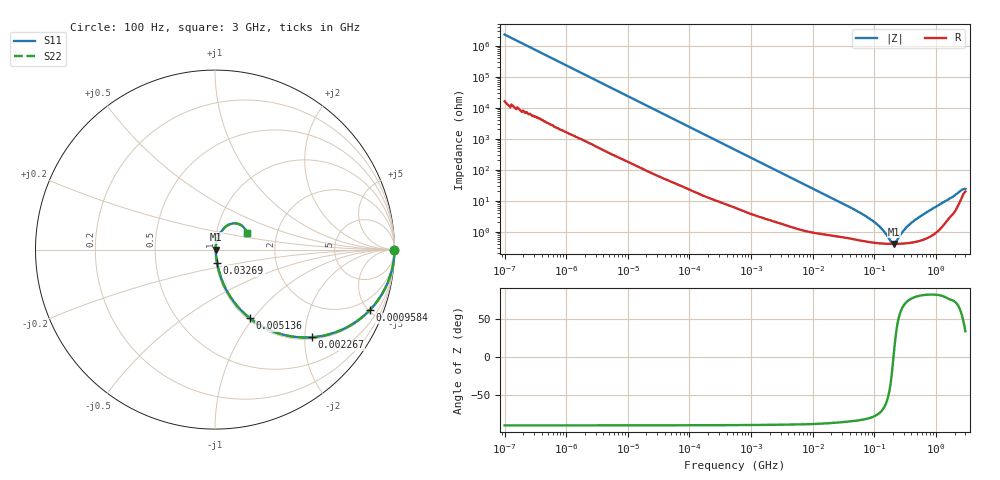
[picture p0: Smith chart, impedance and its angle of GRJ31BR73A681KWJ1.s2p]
!Murata Part Number: GRJ31BR73A681KWJ1
!These Parameters are Measured in Series Mode Connection
!Data Generated on Jun 19, 2026
!  o--ll--o
!Port1  Port2
!  o------o
!Operation Temp=25[degC], DC Bias Voltage=0[V]
!Freq. Start=100[Hz] Stop=3[GHz] 401[Steps]
# Hz S RI R 50
!Freq.(Hz) S11(Real) S11(Imag) S21(Real) S21(Imag) S12(Real) S12(Imag) S22(Real) S22(Imag)
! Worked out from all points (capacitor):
!   401 points, 100 Hz to 3 GHz, reference 50 ohm
!   read as one part in series: C = 684 pF near 109 Hz
!   lowest |Z| = 408 mohm at 208 MHz (marker M1)
!   series resonance near 204.4 MHz, so ESL is about 890 pH
!   S11 on the Smith chart (normalised r, x): 100 Hz: open; 958.4 kHz: 1.08, -5.09; 2.267 MHz: 1.04, -2.17; 5.136 MHz: 1.03, -0.97; 32.69 MHz: 1.01, -0.15; 3 GHz: 1.40, +0.27
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100  1 -4.3e-05  3e-07 4.3e-05  3e-07 4.3e-05  1 -4.3e-05
247  1 -0.000106  7e-07 0.000106  7e-07 0.000106  1 -0.000106
1788  1 -0.00076  6.1e-06 0.00076  6.1e-06 0.00076  1 -0.00076
31977  0.9997 -0.0134  0.000289 0.0134  0.000289 0.0134  0.9997 -0.0134
171338  0.9943 -0.0707  0.00575 0.0707  0.00575 0.0707  0.9943 -0.0707
547723  0.9489 -0.2135  0.051 0.2135  0.051 0.2135  0.9489 -0.2135
958445  0.8624 -0.337  0.1376 0.337  0.1376 0.337  0.8624 -0.337
2266852  0.5394 -0.4884  0.4606 0.4884  0.4606 0.4884  0.5394 -0.4884
5135543  0.1955 -0.3832  0.8045 0.3832  0.8045 0.3832  0.1955 -0.3832
9794414  0.0685 -0.2346  0.9315 0.2346  0.9315 0.2346  0.0685 -0.2346
3.268714e7  0.0122 -0.0748  0.9878 0.0748  0.9878 0.0748  0.0122 -0.0748
1.000898e8  0.00479 -0.0199  0.9952 0.0199  0.9952 0.0199  0.00479 -0.0199
1.352818e8  0.00427 -0.0109  0.9957 0.0109  0.9957 0.0109  0.00427 -0.0109
1.751444e8  0.00407 -0.004  0.9959 0.004  0.9959 0.004  0.00407 -0.004
1.908894e8  0.00405 -0.00177  0.996 0.00177  0.996 0.00177  0.00405 -0.00177
2.080499e8  0.00404 0.000457  0.996 -0.000457  0.996 -0.000457  0.00404 0.000457
2.26753e8  0.00406 0.00269  0.9959 -0.00269  0.9959 -0.00269  0.00406 0.00269
3.199599e8  0.00435 0.012  0.9957 -0.012  0.9957 -0.012  0.00435 0.012
4.713361e8  0.00531 0.0244  0.9947 -0.0244  0.9947 -0.0244  0.00531 0.0244
1.71441e9  0.042 0.109  0.958 -0.109  0.958 -0.109  0.042 0.109
2.525516e9  0.121 0.1455  0.879 -0.1455  0.879 -0.1455  0.121 0.1455
3e9  0.1762 0.0918  0.8238 -0.0918  0.8238 -0.0918  0.1762 0.0918
